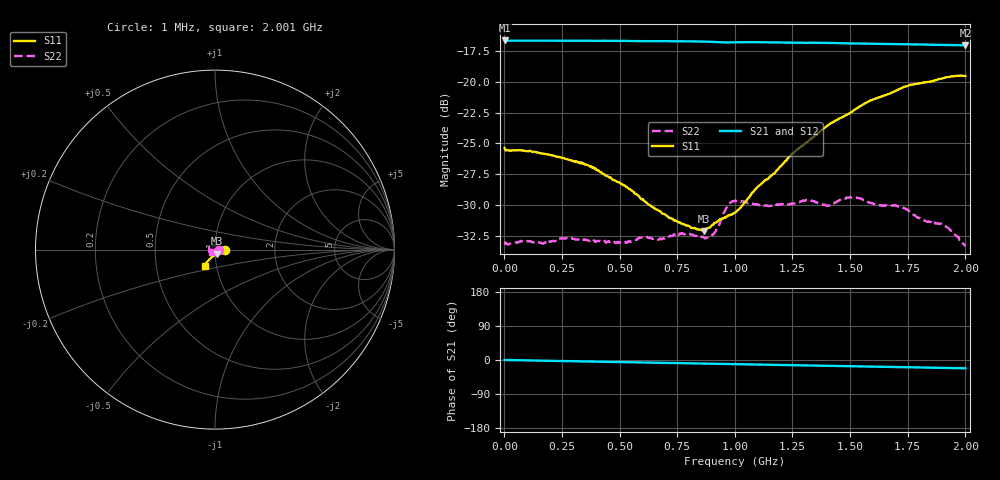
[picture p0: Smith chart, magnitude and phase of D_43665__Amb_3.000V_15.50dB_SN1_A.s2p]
! device id: 43665_
! dir: \\malibu\benchdata\1_engineers\tn_data\43665_75ohm\new\sparar\43665_\amb\3p000v\15p50db
! Serial: 1
! Insertion: A
! Temp: Amb
! VDD: 3.000V
! Attenuation Step: 15.50dB
! IDD: 1.449900e+00mA
! FILE NAME
! DATE 03-27-2009 08:37:10
! CORRECTED  DATA
#  Hz  S  RI  R  75
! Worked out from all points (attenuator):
!   401 points, 1 MHz to 2.001 GHz, reference 75 ohm
!   highest |S21| = -16.62 dB at 1 MHz (marker M1); lowest = -17.0 dB at 2.001 GHz (marker M2)
!   lowest |S11| = -32.1 dB at 866 MHz (marker M3), VSWR 1.05, Z = 76.6 - j3.4 ohm
!   |S11| at or under -10 dB: start of sweep to end of sweep
!   |S22| runs from -33.4 to -29.3 dB; largest |S21 - S12| = 0.00041
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1000000  0.0539 -0.000446  0.1476 -7.06e-05  0.1476 -0.000245  0.0224 -0.000149
1.36e8  0.0519 -0.00143  0.1473 -0.00364  0.1473 -0.00365  0.0207 0.00859
3.36e8  0.0468 -0.00514  0.1469 -0.00918  0.147 -0.00916  0.0135 0.0185
5.26e8  0.0365 -0.00953  0.1462 -0.0145  0.1463 -0.0145  0.00318 0.0221
5.91e8  0.0317 -0.0112  0.1457 -0.0163  0.1458 -0.0163  -0.00201 0.0232
6.71e8  0.0263 -0.0142  0.1455 -0.0185  0.1454 -0.0184  -0.00587 0.0221
7.61e8  0.02 -0.018  0.1449 -0.0212  0.145 -0.0211  -0.0115 0.0213
8.66e8  0.011 -0.0222  0.144 -0.0245  0.144 -0.0244  -0.0177 0.0151
9.06e8  0.00743 -0.0252  0.1433 -0.0257  0.1434 -0.0255  -0.0204 0.0125
9.71e8  0.0026 -0.0285  0.1424 -0.0267  0.1425 -0.0266  -0.0292 0.0123
1.001e9  -0.000233 -0.0295  0.1425 -0.0273  0.1425 -0.0272  -0.03 0.0135
1.096e9  -0.00937 -0.036  0.142 -0.0303  0.1421 -0.0301  -0.0303 0.00976
1.161e9  -0.0141 -0.0393  0.1414 -0.032  0.1416 -0.0319  -0.0306 0.00694
1.256e9  -0.0224 -0.0465  0.1404 -0.0347  0.1405 -0.0346  -0.032 0.00119
1.336e9  -0.0285 -0.052  0.1396 -0.0368  0.1399 -0.0366  -0.0329 -0.002
1.406e9  -0.0338 -0.0578  0.1388 -0.039  0.1391 -0.0389  -0.0308 -0.00612
1.511e9  -0.0406 -0.0642  0.1374 -0.0415  0.1376 -0.0415  -0.0324 -0.00957
1.671e9  -0.0489 -0.075  0.1353 -0.0455  0.1356 -0.0455  -0.0291 -0.0118
1.726e9  -0.0518 -0.0791  0.1346 -0.0468  0.1348 -0.0469  -0.0277 -0.014
1.826e9  -0.0534 -0.0841  0.1333 -0.0489  0.1332 -0.0493  -0.024 -0.013
1.906e9  -0.0565 -0.087  0.1322 -0.0506  0.1323 -0.0506  -0.0228 -0.0131
2.001e9  -0.0566 -0.0894  0.1309 -0.0526  0.1308 -0.0529  -0.0186 -0.0108
